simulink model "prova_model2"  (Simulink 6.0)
settings: Solver=ode45  StartTime=0.0  StopTime=10.0  RelTol=1e-3

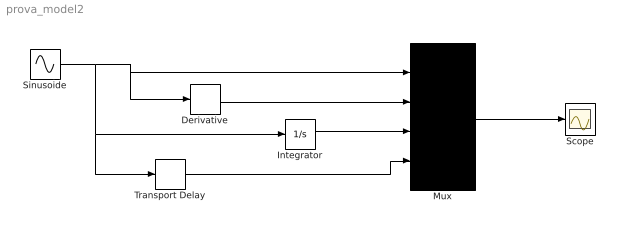
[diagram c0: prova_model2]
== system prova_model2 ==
  Derivative : Derivative
  Integrator : Integrator
  Mux : Mux
  Scope : Scope
  Sinusoide : Sin  SampleTime=0
  Transport Delay : TransportDelay  DelayTime=2
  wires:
  Sinusoide/1 -> Integrator/1, Transport Delay/1, Derivative/1, Mux/1
  Derivative/1 -> Mux/2
  Integrator/1 -> Mux/3
  Transport Delay/1 -> Mux/4
  Mux/1 -> Scope/1
